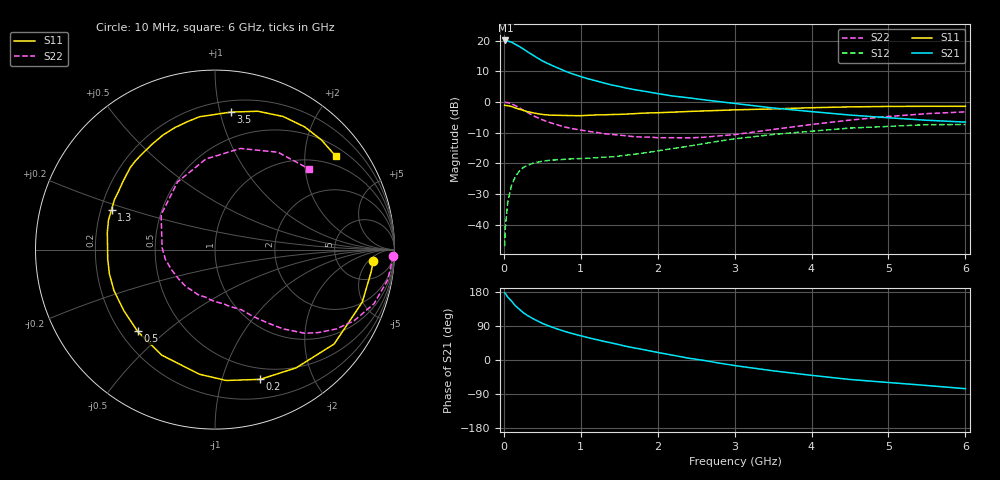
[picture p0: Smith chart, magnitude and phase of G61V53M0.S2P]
! SIEMENS Small Signal Semiconductors
! BFG193
! Si NPN RF Bipolar Junction Transistor in SOT223
! VCE = 1.5 V  IC = 3 mA
! Common Emitter S-Parameters:  August  1996
# GHz  S  MA  R  50
!  f  S11  S21  S12  S22
! GHz  MAG  ANG  MAG  ANG  MAG  ANG  MAG  ANG
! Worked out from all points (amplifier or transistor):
!   36 points, 10 MHz to 6 GHz, reference 50 ohm
!   highest |S21| = 20.0 dB at 20 MHz (marker M1)
!   |S21| within 3 dB of that: start of sweep to 266.6 MHz
!   unconditionally stable (mu >= 1): 1.258 GHz to 2.774 GHz
!   at 250 MHz: K = 0.24, MSG = 19.3 dB, |S12| = -21.4 dB
!   at 1.4 GHz: K = 1.08, MAG = 10.0 dB, |S12| = -17.8 dB
!   at 6 GHz: K = 0.97, MSG = 0.4 dB, |S12| = -7.3 dB
!   S11 on the Smith chart (normalised r, x): 10 MHz: 12, -7; 200 MHz: 0.38, -1.34; 500 MHz: 0.27, -0.40; 1.3 GHz: 0.24, +0.18; 3.5 GHz: 0.29, +1.08; 6 GHz: 0.73, +2.75
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0.01  0.8837 -4.2  9.979 177.1  0.0045 90.7  0.9928 -2.0
0.02  0.879 -8.0  10.04 175.5  0.0092 84.8  0.9879 -3.9
0.05  0.8712 -19.7  9.851 166.3  0.023 79.2  0.9775 -9.9
0.1  0.8469 -38.4  9.405 155.4  0.0441 70.2  0.9357 -18.8
0.15  0.7989 -55.6  8.682 143.1  0.0611 60.5  0.8704 -27.1
0.2  0.7654 -70.8  8.018 134.2  0.0745 53.9  0.8084 -33.1
0.25  0.7319 -85.1  7.338 125.3  0.0854 47.3  0.7392 -38.7
0.3  0.6999 -97.1  6.671 118.2  0.0928 42.8  0.6833 -43.0
0.4  0.6586 -116.8  5.558 106.8  0.1026 35.6  0.5841 -49.2
0.5  0.6272 -133.5  4.678 96.7  0.1087 30.4  0.5134 -53.6
0.6  0.6111 -146.3  4.073 88.6  0.1126 27.5  0.4625 -57.3
0.7  0.6075 -157.9  3.588 81.4  0.1146 25.4  0.4232 -60.8
0.9  0.6001 -175.0  2.848 69.2  0.119 23.2  0.3667 -66.3
1.1  0.6076 170.9  2.377 58.8  0.1215 22.9  0.3335 -73.7
1.3  0.6178 158.9  2.044 49.3  0.1262 23.7  0.3054 -80.9
1.6  0.6364 144.1  1.674 35.7  0.1368 25.1  0.2812 -94.9
2.2  0.6835 121.0  1.25 12.5  0.175 25.4  0.2624 -128.6
2.8  0.7292 102.1  1.014 -8.1  0.2309 19.4  0.2813 -168.6
3.5  0.7713 83.4  0.799 -28.5  0.296 5.0  0.3577 147.1
4.5  0.8331 62.9  0.613 -51.4  0.3766 -16.1  0.5072 95.8
5.5  0.8515 45.8  0.504 -67.3  0.4281 -41.8  0.6461 57.1
6  0.8503 37.8  0.471 -75.7  0.43 -56.0  0.6913 40.4
